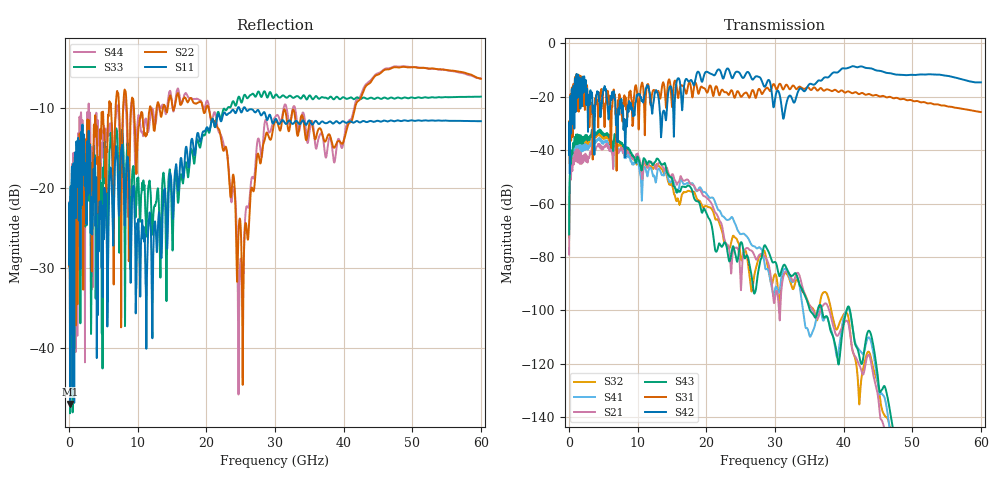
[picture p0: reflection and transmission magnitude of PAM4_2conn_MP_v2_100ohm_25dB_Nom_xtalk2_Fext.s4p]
! Info: Touchstone file created by Circ.  Input file=FAB50GbE_2conn_Midplane_Examax_Topo2_v2_100ohm_25dB_Nom.circ
# Hz S RI R 50
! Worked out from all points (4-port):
!   6000 points, 10 MHz to 60 GHz, reference 50 ohm
!   strongest paths, dB at 10 MHz, 15.01 GHz, 30.01 GHz, 45.01 GHz, 60 GHz:
!     S42: -41.7, -18.2, -20.8, -10.2, -14.6
!     S31: -41.3, -23.8, -16.0, -19.6, -25.7
!     S43: -71.5, -50.7, -81.8, -125.3, -173.3
!     S21: -79.0, -49.0, -95.2, -132.2, -178.9
!     S41: -71.1, -50.5, -92.0, -127.6, -183.8
!     S32: -72.8, -52.9, -86.4, -127.5, -175.7
!   lowest |S11| = -47.0 dB at 140 MHz (marker M1), VSWR 1.01, Z = 49.7 + j0.366 ohm
!   |S11| at or under -10 dB: start of sweep to 24.61 GHz; 24.79 GHz to 25.43 GHz (644.5 MHz wide, 2.57 % of centre); 25.63 GHz to end of sweep
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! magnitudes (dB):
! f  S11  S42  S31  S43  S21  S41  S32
! 10 MHz  -29.6  -41.7  -41.3  -71.5  -79.0  -71.1  -72.8
! 140 MHz  -47.0  -28.4  -27.4  -46.9  -51.8  -48.5  -49.0
! 5.5 GHz  -27.2  -20.6  -19.5  -33.7  -38.1  -36.5  -35.0
! 23.37 GHz  -10.7  -10.4  -18.9  -81.6  -77.7  -65.9  -76.7
! 24.87 GHz  -10.2  -11.1  -19.2  -75.9  -82.7  -71.2  -76.9
! 28.66 GHz  -11.0  -15.7  -16.9  -76.0  -80.4  -84.6  -79.7
! 60 GHz  -11.7  -14.6  -25.7  -173.3  -178.9  -183.8  -175.7
